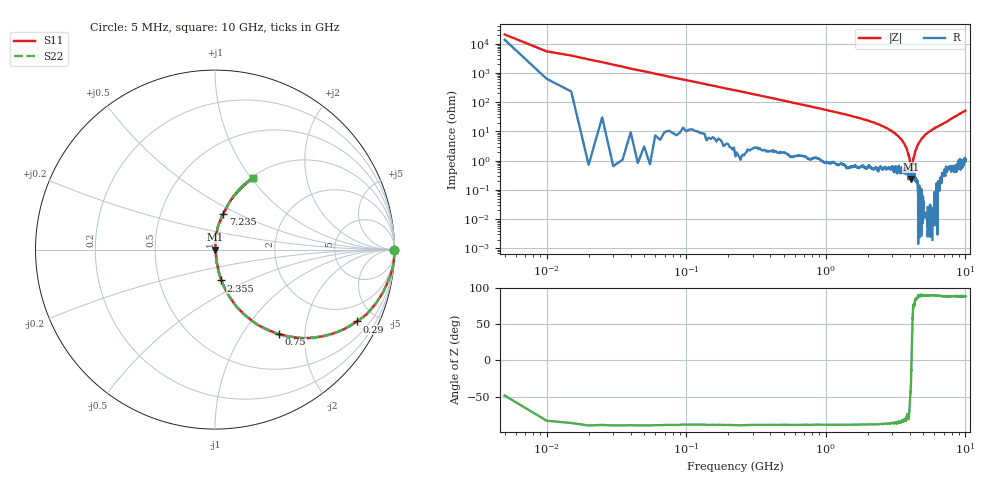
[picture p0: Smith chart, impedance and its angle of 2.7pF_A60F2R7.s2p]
! Amotech Co.,Ltd.
! http://www.amotech.co.kr/
! Part Number: A60F2R7
! These Parameters are Measured in Series Mode Connection
! Operation Temp=25[degC], DC Bias Voltage=0[V]
! Freq. Start=5[MHz] Stop=10[GHz], 2000[Steps]
! Date: Monday, July 20, 2020, 03:20:59
# GHZ S RI R 50.000000
!Freq.(Hz) S11(Real) S11(Imag) S21(Real) S21(Imag) S12(Real) S12(Imag) S22(Real) S22(Imag)
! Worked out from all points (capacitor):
!   2000 points, 5 MHz to 10 GHz, reference 50 ohm
!   read as one part in series: C = 2.82 pF near 55 MHz
!   lowest |Z| = 236 mohm at 4.09 GHz (marker M1)
!   series resonance near 4.108 GHz, so ESL is about 530 pH
!   S11 on the Smith chart (normalised r, x): 5 MHz: open; 290 MHz: 1.05, -3.93; 750 MHz: 1.02, -1.48; 2.355 GHz: 1.01, -0.36; 7.235 GHz: 1.01, +0.41; 10 GHz: 1.02, +1.02
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0.005  0.9968 -0.00361  0.0032 0.00361  0.0032 0.00361  0.9968 -0.00361
0.06  0.9881 -0.1047  0.0119 0.1047  0.0119 0.1047  0.9881 -0.1047
0.09  0.9731 -0.1549  0.0269 0.1549  0.0269 0.1549  0.9731 -0.1549
0.17  0.914 -0.272  0.086 0.272  0.086 0.272  0.914 -0.272
0.29  0.791 -0.4004  0.209 0.4004  0.209 0.4004  0.791 -0.4004
0.75  0.357 -0.4711  0.643 0.4711  0.643 0.4711  0.357 -0.4711
1.145  0.1857 -0.3793  0.8143 0.3793  0.8143 0.3793  0.1857 -0.3793
1.675  0.0873 -0.2724  0.9127 0.2724  0.9127 0.2724  0.0873 -0.2724
2.355  0.035 -0.1716  0.965 0.1716  0.965 0.1716  0.035 -0.1716
3.34  0.0107 -0.0633  0.9893 0.0633  0.9893 0.0633  0.0107 -0.0633
3.805  0.0062 -0.0246  0.9938 0.0246  0.9938 0.0246  0.0062 -0.0246
3.975  0.00488 -0.0112  0.9951 0.0112  0.9951 0.0112  0.00488 -0.0112
4.09  0.00222 -0.000766  0.9978 0.000766  0.9978 0.000766  0.00222 -0.000766
4.13  0.00355 0.00103  0.9965 -0.00103  0.9965 -0.00103  0.00355 0.00103
4.235  0.0029 0.0112  0.9971 -0.0112  0.9971 -0.0112  0.0029 0.0112
4.39  0.00271 0.0219  0.9973 -0.0219  0.9973 -0.0219  0.00271 0.0219
4.675  0.00288 0.043  0.9971 -0.043  0.9971 -0.043  0.00288 0.043
5.005  0.00481 0.0662  0.9952 -0.0662  0.9952 -0.0662  0.00481 0.0662
6.67  0.0297 0.1626  0.9703 -0.1626  0.9703 -0.1626  0.0297 0.1626
7.235  0.0456 0.1962  0.9544 -0.1962  0.9544 -0.1962  0.0456 0.1962
8.335  0.0953 0.2842  0.9047 -0.2842  0.9047 -0.2842  0.0953 0.2842
10  0.213 0.3986  0.787 -0.3986  0.787 -0.3986  0.213 0.3986
